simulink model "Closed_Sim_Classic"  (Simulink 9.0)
settings: Solver=ode45  StartTime=0.0  StopTime=60  RelTol=1e-3  EnableMultiTasking=on
InitFcn:
  | init
StartFcn:
  | init
StopFcn:
  | pl
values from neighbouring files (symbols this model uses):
  d2r = 1/r2d    (= 0.0174532925199)    [init.m]    (also in freq.m; frequ.m; init_lat.m; pl.m)
  r2d = 180/pi    (= 57.2957795131)    [init.m]    (also in freq.m; frequ.m; init_lat.m; pl.m)
undefined symbols (not defined in the file or in its folder): Av, Bv, Cv, Dv

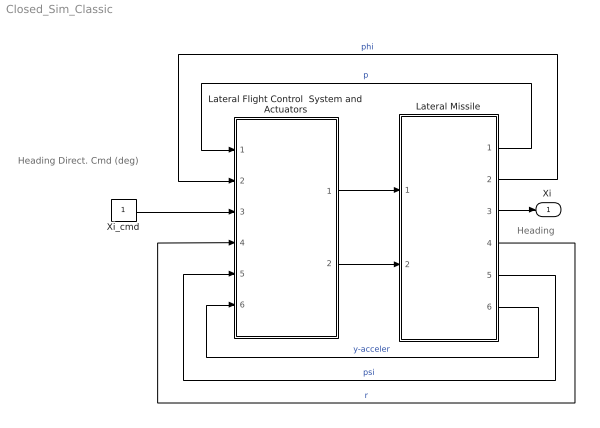
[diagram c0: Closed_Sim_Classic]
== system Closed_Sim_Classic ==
  note: Heading Direct. Cmd (deg)
  note: Heading
  Lateral Flight Control  System and Actuators : Subsystem
  Lateral Missile : Subsystem
  Xi_cmd : Constant
  "Xi " : Outport
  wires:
  Lateral Flight Control  System and Actuators/1(d-ailer) -> Lateral Missile/1(dail)
  Lateral Flight Control  System and Actuators/2(d-ruddr) -> Lateral Missile/2(drud)
  Lateral Missile/6(Ny) -> Lateral Flight Control  System and Actuators/6(Nym)  "y-acceler"
  Lateral Missile/5(psi) -> Lateral Flight Control  System and Actuators/5(psi)  "psi"
  Lateral Missile/4(r) -> Lateral Flight Control  System and Actuators/4(r)  "r"
  Lateral Missile/1(p) -> Lateral Flight Control  System and Actuators/1(p)  "p"
  Lateral Missile/2(phi) -> Lateral Flight Control  System and Actuators/2(phi)  "phi"
  Lateral Missile/3("Xi ") -> "Xi "/1
  Xi_cmd/1 -> Lateral Flight Control  System and Actuators/3(Xi_cmd)

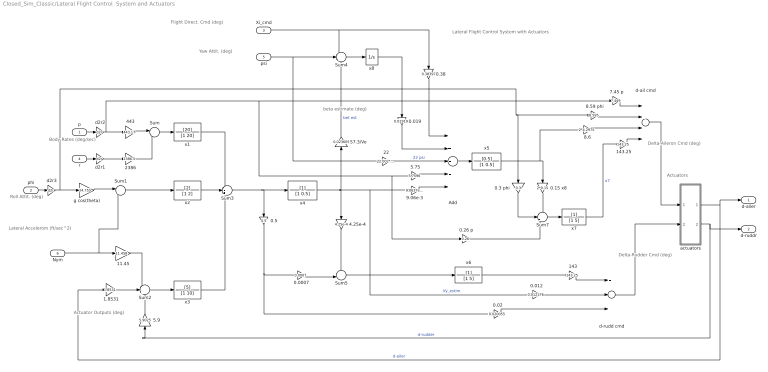
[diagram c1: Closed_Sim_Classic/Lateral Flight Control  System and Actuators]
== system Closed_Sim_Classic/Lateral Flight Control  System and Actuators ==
  note: Body Rates (deg/sec)
  note: Delta-Rudder Cmd (deg)
  note: Delta-Aileron Cmd (deg)
  note: Lateral Accelerom (ft/sec^2)
  note: Actuator Outputs (deg)
  note: Roll Attit. (deg)
  note: Yaw Attit. (deg)
  note: Flight Direct. Cmd (deg)
  note: beta estimate (deg)
  note: Actuators
  note: Lateral Flight Control System with Actuators
  p : Inport
  phi : Inport  Port=2
  Xi_cmd : Inport  Port=3
  r : Inport  Port=4
  psi : Inport  Port=5
  Nym : Inport  Port=6
  0.0007 : Gain  Gain=0.0007
  0.012 : Gain  Gain=0.012176
  0.019 : Gain  Gain=0.019199
  0.02 : Gain  Gain=0.020055
  0.15 x8 : Gain  Gain=2*0.15
  0.26 p : Gain  Gain=0.26
  0.3 phi : Gain  Gain=0.3
  0.38 : Gain  Gain=0.38397
  0.5 : Gain  Gain=0.5
  1.8531 : Gain  Gain=1.8531
  11.45 : Gain  Gain=11.458
  143 : Gain  Gain=143.25
  143.25 : Gain  Gain=143.25
  22 : Gain  Gain=22.002*d2r
  2386 : Gain  Gain=2386.5
  4.25e-4 : Gain  Gain=4.25e-4
  443 : Gain  Gain=443.17
  5.75 : Gain  Gain=5.7596
  5.9 : Gain  Gain=5.9025
  57.3/Vo : Gain  Gain=0.023605
  7.45 p : Gain  Gain=7.449
  8.59 phi : Gain  Gain=8.595
  8.6 : Gain  Gain=2*4.2975
  "9.06e-3 " : Gain  Gain=9.0637e-3
  Add : Sum  Inputs=++---
  Sum : Sum  Inputs=|-+
  Sum1 : Sum  Inputs=|++
  Sum2 : Sum  Inputs=-++
  Sum3 : Sum  Inputs=-++
  Sum4 : Sum  Inputs=+--
  Sum5 : Sum  Inputs=--|
  Sum7 : Sum  Inputs=-++
  actuators : Subsystem
  d-ail cmd : Sum  Inputs=++-+
  d-rudd cmd : Sum  Inputs=+--
  d2r1 : Gain  Gain=d2r
  d2r2 : Gain  Gain=d2r
  d2r3 : Gain  Gain=d2r
  g cos(theta) : Gain  Gain=24.755
  x1 : TransferFcn  Numerator=[20]  Denominator=[1 20]
  x2 : TransferFcn  Numerator=[2]  Denominator=[1 2]
  x3 : TransferFcn  Numerator=[5]  Denominator=[1 10]
  x4 : TransferFcn  Denominator=[1 0.5]
  x5 : TransferFcn  Numerator=[0.5]  Denominator=[1 0.5]
  x6 : TransferFcn  Denominator=[1 5]
  x7 : TransferFcn  Denominator=[1 5]
  x8 : Integrator
  d-ailer : Outport
  d-ruddr : Outport  Port=2
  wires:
  0.5/1 -> 0.02/1, 0.0007/1
  d-rudd cmd/1 -> actuators/2(dr)
  0.02/1 -> d-rudd cmd/3
  0.012/1 -> d-rudd cmd/2
  x6/1 -> 143/1
  143/1 -> d-rudd cmd/1
  d-ail cmd/1 -> actuators/1(da)
  7.45 p/1 -> d-ail cmd/1
  8.59 phi/1 -> d-ail cmd/2
  143.25/1 -> d-ail cmd/4
  x7/1 -> 143.25/1  "x7"
  8.6/1 -> d-ail cmd/3
  0.3 phi/1 -> Sum7/2
  0.26 p/1 -> Sum7/3
  0.15 x8/1 -> Sum7/1
  Sum7/1 -> x7/1
  x5/1 -> 8.6/1, 0.15 x8/1
  5.75/1 -> Add/4
  2386/1 -> Add/3  "22 psi"
  0.019/1 -> Add/2
  x8/1 -> 0.019/1
  Add/1 -> x5/1
  "9.06e-3 "/1 -> Add/5
  0.38/1 -> Add/1
  Sum5/1 -> x6/1
  0.0007/1 -> Sum5/2
  4.25e-4/1 -> Sum5/1
  Nym/1 -> Sum1/2, 11.45/1
  Sum4/1 -> x8/1
  57.3/Vo/1 -> Sum4/3  "bet est"
  x4/1 -> 0.012/1, "9.06e-3 "/1, 4.25e-4/1, 57.3/Vo/1  "Vy_estim"
  psi/1 -> Sum4/2, 2386/1
  Xi_cmd/1 -> 0.38/1, Sum4/1
  Sum3/1 -> 0.5/1, x4/1
  x3/1 -> Sum3/3
  x2/1 -> Sum3/2
  x1/1 -> Sum3/1
  Sum2/1 -> x3/1
  5.9/1 -> Sum2/3
  1.8531/1 -> Sum2/2
  11.45/1 -> Sum2/1
  phi/1 -> d2r3/1
  g cos(theta)/1 -> Sum1/1
  Sum1/1 -> x2/1
  2386/1 -> Sum/2
  r/1 -> d2r1/1
  p/1 -> d2r2/1
  443/1 -> Sum/1
  Sum/1 -> x1/1
  actuators/1("da ") -> d-ailer/1, 1.8531/1  "d-ailer"
  actuators/2("dr ") -> d-ruddr/1, 5.9/1  "d-rudder"
  d2r3/1 -> 8.59 phi/1, 0.3 phi/1, g cos(theta)/1
  d2r2/1 -> 7.45 p/1, 0.26 p/1, 5.75/1, 443/1
  d2r1/1 -> 2386/1

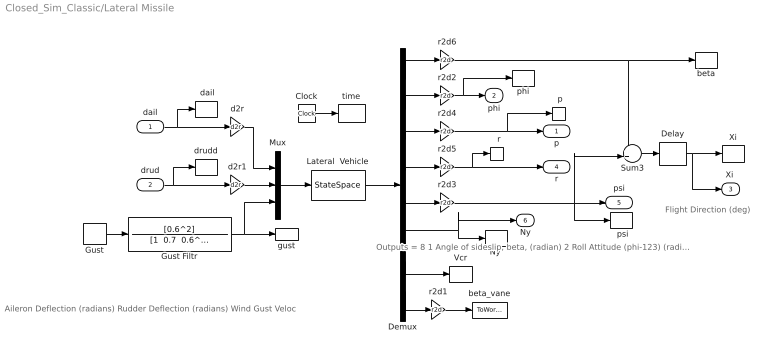
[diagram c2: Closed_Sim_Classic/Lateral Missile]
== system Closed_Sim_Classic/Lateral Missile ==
  note: Aileron Deflection (radians) Rudder Deflection (radians) Wind Gust Veloc
  note: Flight Direction (deg)
  note: Outputs = 8 1 Angle of sideslip, beta, (radian) 2 Roll Attitude (phi-123) (radians) 3 Roll Rate (p-body) (rad/sec) 4 Yaw Rate (r-body) (rad/sec) 5 Yaw Attitude (psi-123) (radians) 6 Y-Acceleromet, (ft/sec^2) Translation 7 Cross Range Velocity (Vcr) (ft/sec) 8 Beta Sensed at Vane # 1 (radian)
  dail : Inport
  drud : Inport  Port=2
  "  r" : ToWorkspace  VariableName=r  SampleTime=-1
  " Xi " : ToWorkspace  VariableName=Xi  SampleTime=-1
  " dail" : ToWorkspace  VariableName=dail  SampleTime=-1
  " drudd " : ToWorkspace  VariableName=drud  SampleTime=-1
  " p" : ToWorkspace  VariableName=p  SampleTime=-1
  " phi " : ToWorkspace  VariableName=phi  SampleTime=-1
  " psi" : ToWorkspace  VariableName=psi  SampleTime=-1
  Clock : Clock
  Delay : TransportDelay  DelayTime=0.7  PadeOrder=2
  Demux : Demux  Outputs=8
  Gust : DiscretePulseGenerator  PulseType=Time based  Amplitude=30  Period=500  PulseWidth=2  PhaseDelay=20
  Gust Filtr : TransferFcn  Numerator=[0.6^2]  Denominator="[1  0.7  0.6^2]"
  Lateral  Vehicle : StateSpace  A=Av  B=Bv  C=Cv  D=Dv  InitialCondition=0
  Mux : Mux  Inputs=3
  "Ny " : ToWorkspace  VariableName=Ny  SampleTime=-1
  Sum3 : Sum  Inputs=++|
  Vcr : ToWorkspace  VariableName=Vcr  SampleTime=-1
  beta : ToWorkspace  VariableName=beta  SampleTime=-1
  beta_vane : ToWorkspace  VariableName=beta_vn  SampleTime=-1
  d2r : Gain  Gain=d2r
  d2r1 : Gain  Gain=d2r
  gust : ToWorkspace  VariableName=Vgst  SampleTime=-1
  r2d{1..6} (6 alike) : Gain  Gain=r2d
  time : ToWorkspace  VariableName=time  SampleTime=-1
  p : Outport
  phi : Outport  Port=2
  "Xi " : Outport  Port=3
  r : Outport  Port=4
  psi : Outport  Port=5
  Ny : Outport  Port=6
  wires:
  Mux/1 -> Lateral  Vehicle/1
  Lateral  Vehicle/1 -> Demux/1
  dail/1 -> d2r/1, " dail"/1
  drud/1 -> d2r1/1, " drudd "/1
  Sum3/1 -> Delay/1
  Demux/1 -> r2d6/1
  Demux/2 -> r2d2/1
  Demux/3 -> r2d4/1
  Demux/4 -> r2d5/1
  Demux/5 -> r2d3/1
  Demux/6 -> Ny/1, "Ny "/1
  r2d2/1 -> phi/1, " phi "/1
  r2d3/1 -> psi/1, Sum3/2, " psi"/1
  r2d4/1 -> p/1, " p"/1
  r2d5/1 -> r/1, "  r"/1
  Gust Filtr/1 -> Mux/3, gust/1
  d2r/1 -> Mux/1
  d2r1/1 -> Mux/2
  Demux/7 -> Vcr/1
  Demux/8 -> r2d1/1
  r2d1/1 -> beta_vane/1
  Clock/1 -> time/1
  r2d6/1 -> beta/1, Sum3/1
  Gust/1 -> Gust Filtr/1
  Delay/1 -> "Xi "/1, " Xi "/1

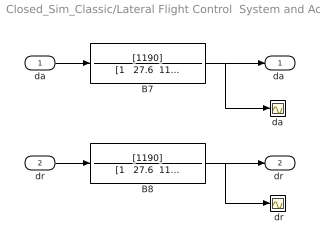
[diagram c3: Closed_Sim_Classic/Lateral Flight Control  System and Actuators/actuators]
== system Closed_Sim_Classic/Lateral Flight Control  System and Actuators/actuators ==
  da : Inport
  dr : Inport  Port=2
  " da " : Scope
  " dr" : Scope
  B7 : TransferFcn  Numerator=[1190]  Denominator="[1   27.6  1190]"
  B8 : TransferFcn  Numerator=[1190]  Denominator="[1   27.6  1190]"
  "da " : Outport
  "dr " : Outport  Port=2
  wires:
  B8/1 -> " dr"/1, "dr "/1
  dr/1 -> B8/1
  B7/1 -> " da "/1, "da "/1
  da/1 -> B7/1
